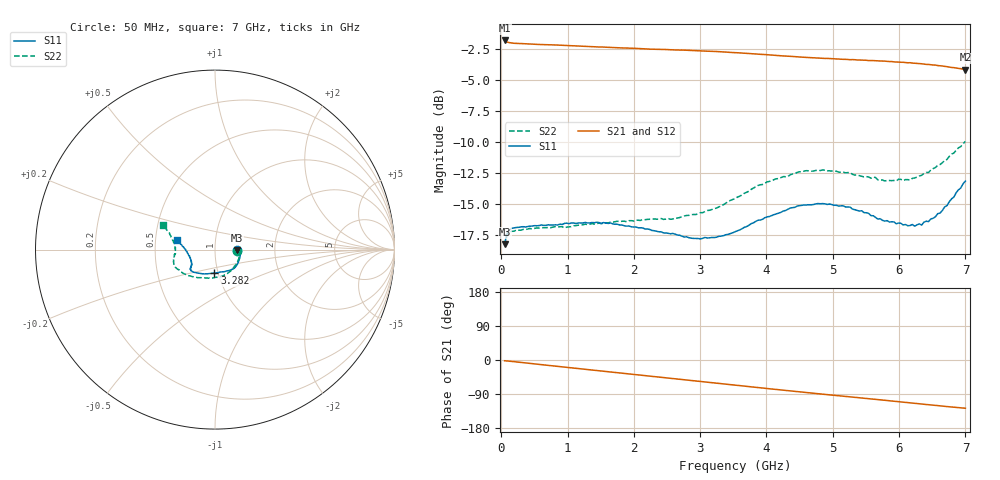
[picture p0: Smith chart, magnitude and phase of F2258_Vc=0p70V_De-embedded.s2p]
! Integrated Device Technology
! Corporate Headquarters
! 6024 Silver Creek Valley Road
! San Jose, CA 95138  USA
! Phone:  1-408-284-8200
! Toll Free:  1-800-223-1366
! Webpage:  http://www.idt.com/
! Timing and RF Division
! 515 Groton Road, Suite 102
! Westford, MA 01886-6024
! Device:  F2258
! Description: Voltage Variable RF Attenuator
! Frequency:  50.0 -  6000.00 MHz
! Package:  3x3 mm Thin QFN Plastic Package: 16 pin
! Ports:  2 RF, 2 DC
!  Pin  1  = NC
!  Pin  2  = NC
!  Pin  3  = RF2  = Port 2
!  Pin  4  = GND
!  Pin  5  = Vdd
!  Pin  6  = NC
!  Pin  7  = VCTRL
!  Pin  8  = NC
!  Pin  9  = GND
!  Pin 10  = RF1  = Port 1
!  Pin 11  = NC
!  Pin 12  = NC
!  Pin 13  = NC
!  Pin 14  = NC
!  Pin 15  = NC
!  Pin 16  = NC
! Vcntrl:  0.700 Volts
! Vdd:  +3.300 Volts
! Current:  1.120 mA
! Data:  The device was measured on a the F2258 evaluation board which has
!  individual transmission lines to the RF pins.  Data was collected
!  using a calibrated network analyzer.  The evaluation board was
!  de-embedded using a TRL calibration technique.
!  The reference plane is the edge of the package pin.
! Misc:  SN 10
!  Action Tracker AT0285
! Date Measured:  2014-12-10
! Date:  2016-01-13  MJV
! Note:
!  Integrated Device Technology supplies this data as a sample of measured
!  data at the package pin for this product.  Your particular data for this
!  product may vary.
!  Data was taken at 25 degrees C.
!  Integrated Device Technology reserves the right to change this data at anytime.
!Freq_(GHz)  S11M_(dB)  S11P_(deg)  S21M_(dB)  S21P_(deg)  S12M_(dB)  S12P_(deg)  S22M_(dB)  S22P_(deg)
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# GHz S dB R 50
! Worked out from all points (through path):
!   201 points, 50 MHz to 7 GHz, reference 50 ohm
!   highest |S21| = -1.82 dB at 50 MHz (marker M1); lowest = -4.2 dB at 7 GHz (marker M2)
!   group delay of S21, straight-line fit = 50.4 ps
!   lowest |S11| = -18.3 dB at 50 MHz (marker M3), VSWR 1.28, Z = 63.9 - j0.516 ohm
!   |S11| at or under -10 dB: start of sweep to end of sweep
!   |S22| runs from -18.4 to -10.0 dB; largest |S21 - S12| = 0.0018
!   S11 on the Smith chart (normalised r, x): 50 MHz: 1.28, -0.01; 3.282 GHz: 0.96, -0.26; 7 GHz: 0.65, +0.08
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0.05  -18.28 -1.9  -1.82 -2.0  -1.82 -2.0  -18.42 -2.6
0.08475  -17.40 -3.1  -1.94 -2.5  -1.95 -2.5  -17.55 -3.9
0.15425  -16.98 -5.0  -2.02 -3.7  -2.02 -3.7  -17.22 -6.9
0.77975  -16.71 -24.2  -2.18 -15.5  -2.18 -15.5  -16.88 -31.9
0.9535  -16.58 -30.2  -2.22 -18.8  -2.21 -18.8  -16.96 -39.6
1.2315  -16.55 -37.1  -2.29 -24.0  -2.28 -24.0  -16.69 -49.4
1.6485  -16.55 -45.8  -2.38 -31.6  -2.38 -31.6  -16.49 -62.2
2.37825  -17.26 -59.5  -2.54 -44.8  -2.53 -44.8  -16.23 -82.0
2.58675  -17.40 -64.9  -2.57 -48.7  -2.57 -48.6  -16.23 -88.5
2.8995  -17.79 -75.4  -2.64 -54.5  -2.63 -54.5  -15.86 -99.4
3.28175  -17.63 -91.4  -2.72 -61.7  -2.71 -61.7  -15.25 -114.9
3.525  -17.27 -102.6  -2.80 -66.3  -2.78 -66.3  -14.58 -124.5
4.0115  -16.06 -122.5  -2.97 -75.3  -2.96 -75.3  -13.23 -141.5
4.46325  -15.19 -133.9  -3.14 -83.5  -3.13 -83.5  -12.47 -153.7
4.7065  -15.07 -137.2  -3.22 -87.7  -3.21 -87.7  -12.36 -158.4
5.2625  -15.27 -143.1  -3.37 -97.3  -3.38 -97.3  -12.49 -167.5
5.85325  -16.47 -150.2  -3.52 -107.5  -3.52 -107.5  -13.12 -178.6
6.166  -16.75 -158.4  -3.62 -113.1  -3.62 -113.0  -13.09 174.6
6.2355  -16.81 -161.9  -3.66 -114.2  -3.66 -114.2  -12.91 172.6
6.444  -16.44 -171.0  -3.75 -118.0  -3.76 -118.0  -12.47 167.6
6.722  -15.15 175.5  -3.93 -122.8  -3.93 -122.8  -11.43 160.2
7  -13.17 165.2  -4.17 -127.3  -4.18 -127.3  -9.97 154.7
